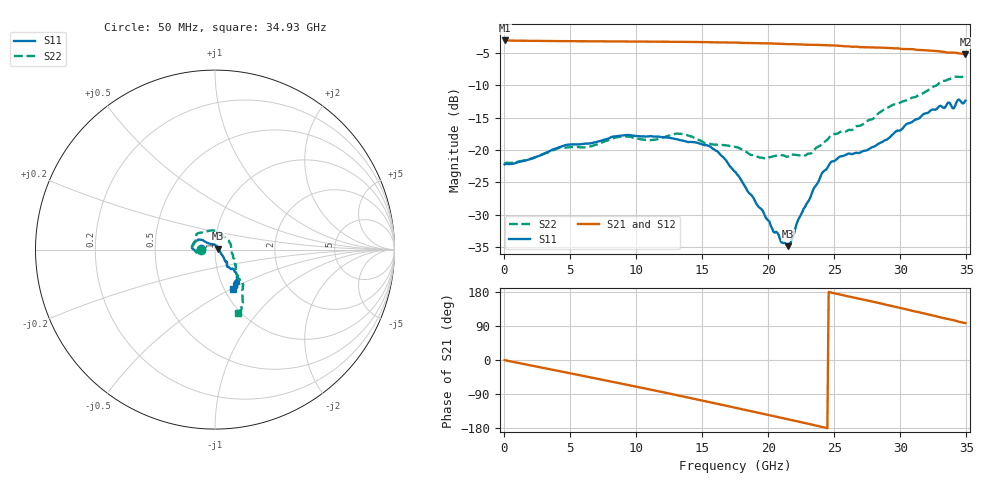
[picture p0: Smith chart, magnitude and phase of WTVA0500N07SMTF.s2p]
! 50 ohm 2-Port S-parameters measured by Modelithics Inc support@modelithics.com  Tampa, FL USA 813-866-6335 (February 2024)
! Smiths Interconnect,  5dB P/N: WTVA0500N07SMTF, Temperature: 125 C
! Board: 10 mil Rogers 4350B, Mounting Pad Dimensions: Length: 15 mils, Width: 25 mils, Gap: 40 mils.
# Hz S RI R 50
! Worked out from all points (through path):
!   352 points, 50 MHz to 34.93 GHz, reference 50 ohm
!   highest |S21| = -3.06 dB at 50 MHz (marker M1); lowest = -5.2 dB at 34.93 GHz (marker M2)
!   group delay of S21, straight-line fit = 20.9 ps
!   lowest |S11| = -34.9 dB at 21.49 GHz (marker M3), VSWR 1.04, Z = 51.8 + j0.464 ohm
!   |S11| at or under -10 dB: start of sweep to end of sweep
!   |S22| runs from -22.1 to -8.5 dB; largest |S21 - S12| = 0.0085
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5e7  -0.0774 0.000955  0.7031 -0.00431  0.7022 -0.00408  -0.0783 -0.000842
2.787e9  -0.0911 -0.00339  0.6568 -0.2338  0.6557 -0.2339  -0.0911 -0.00713
4.18e9  -0.1045 -0.0104  0.6063 -0.3395  0.6051 -0.3393  -0.1026 -0.0158
5.8715e9  -0.1108 -0.00596  0.5229 -0.456  0.5221 -0.4556  -0.1041 -0.0108
8.8565e9  -0.1287 0.0122  0.3234 -0.6101  0.3213 -0.6099  -0.1264 0.0121
1.1742e10  -0.1232 0.0291  0.0861 -0.682  0.0844 -0.6811  -0.1063 0.0609
1.3334e10  -0.11 0.0455  -0.0541 -0.6842  -0.0557 -0.683  -0.0998 0.0886
1.5523e10  -0.092 0.0551  -0.2434 -0.6365  -0.2456 -0.6342  -0.0477 0.1013
1.7513e10  -0.0528 0.0424  -0.3978 -0.5477  -0.3978 -0.5462  -0.00167 0.1057
1.98015e10  -0.00917 0.0287  -0.5363 -0.3979  -0.5358 -0.3968  0.0558 0.0649
2.09955e10  0.0128 0.0145  -0.5886 -0.3035  -0.5879 -0.3026  0.0784 0.0465
2.1493e10  0.0175 0.00448  -0.6024 -0.2644  -0.602 -0.2625  0.0802 0.0383
2.33835e10  0.0384 -0.0298  -0.6428 -0.1015  -0.6419 -0.1012  0.0944 -0.021
2.47765e10  0.0556 -0.0592  -0.6437 0.0237  -0.6428 0.0253  0.1126 -0.0661
2.63685e10  0.0641 -0.0675  -0.6086 0.1554  -0.6072 0.1567  0.1125 -0.0883
2.91545e10  0.0771 -0.0973  -0.4978 0.3611  -0.493 0.3657  0.1375 -0.1659
3.23385e10  0.1252 -0.1609  -0.2796 0.5146  -0.2753 0.5156  0.1529 -0.2599
3.33335e10  0.1187 -0.1744  -0.1963 0.538  -0.1924 0.5384  0.1459 -0.3097
3.3632e10  0.1277 -0.1951  -0.1744 0.5387  -0.169 0.5397  0.1465 -0.3202
3.403e10  0.113 -0.176  -0.1479 0.546  -0.1423 0.5466  0.1441 -0.3364
3.43285e10  0.1142 -0.2131  -0.1173 0.5488  -0.1134 0.5487  0.1357 -0.3428
3.49255e10  0.1011 -0.2185  -0.0707 0.5441  -0.0693 0.543  0.1287 -0.3517
